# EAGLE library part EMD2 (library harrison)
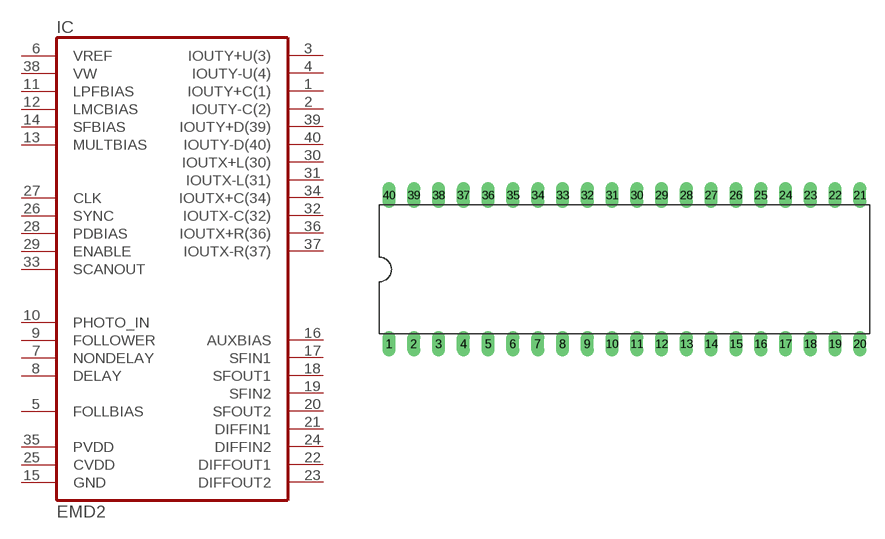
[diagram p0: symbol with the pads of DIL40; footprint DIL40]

Designator prefix IC

## EMD2  [DIL40]
1  IOUTY+C(1)  out
2  IOUTY-C(2)  out
3  IOUTY+U(3)  out
4  IOUTY-U(4)  out
5  FOLLBIAS  in
6  VREF  in
7  NONDELAY  out
8  DELAY  out
9  FOLLOWER  out
10  PHOTO_IN  in
11  LPFBIAS  in
12  LMCBIAS  in
13  MULTBIAS  in
14  SFBIAS  in
15  GND  pwr
16  AUXBIAS  in
17  SFIN1  in
18  SFOUT1  out
19  SFIN2  in
20  SFOUT2  out
21  DIFFIN1  in
22  DIFFOUT1  out
23  DIFFOUT2  out
24  DIFFIN2  in
25  CVDD  pwr
26  SYNC  out
27  CLK  in
28  PDBIAS  in
29  ENABLE  in
30  IOUTX+L(30)  out
31  IOUTX-L(31)  out
32  IOUTX-C(32)  out
33  SCANOUT  out
34  IOUTX+C(34)  out
35  PVDD  pwr
36  IOUTX+R(36)  out
37  IOUTX-R(37)  out
38  VW  in
39  IOUTY+D(39)  out
40  IOUTY-D(40)  out

## Footprint DIL40 (pad centres in mm)
drill 0.813 long: 1 -22.86,-7.62; 2 -20.32,-7.62; 3 -17.78,-7.62; 4 -15.24,-7.62; 5 -12.7,-7.62; 6 -10.16,-7.62; 7 -7.62,-7.62; 8 -5.08,-7.62; 9 -2.54,-7.62; 10 0,-7.62; 11 2.54,-7.62; 12 5.08,-7.62; 13 7.62,-7.62; 14 10.16,-7.62; 15 12.7,-7.62; 16 15.24,-7.62; 17 17.78,-7.62; 18 20.32,-7.62; 19 22.86,-7.62; 20 25.4,-7.62; 21 25.4,7.62; 22 22.86,7.62; 23 20.32,7.62; 24 17.78,7.62; 25 15.24,7.62; 26 12.7,7.62; 27 10.16,7.62; 28 7.62,7.62; 29 5.08,7.62; 30 2.54,7.62; 31 0,7.62; 32 -2.54,7.62; 33 -5.08,7.62; 34 -7.62,7.62; 35 -10.16,7.62; 36 -12.7,7.62; 37 -15.24,7.62; 38 -17.78,7.62; 39 -20.32,7.62; 40 -22.86,7.62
